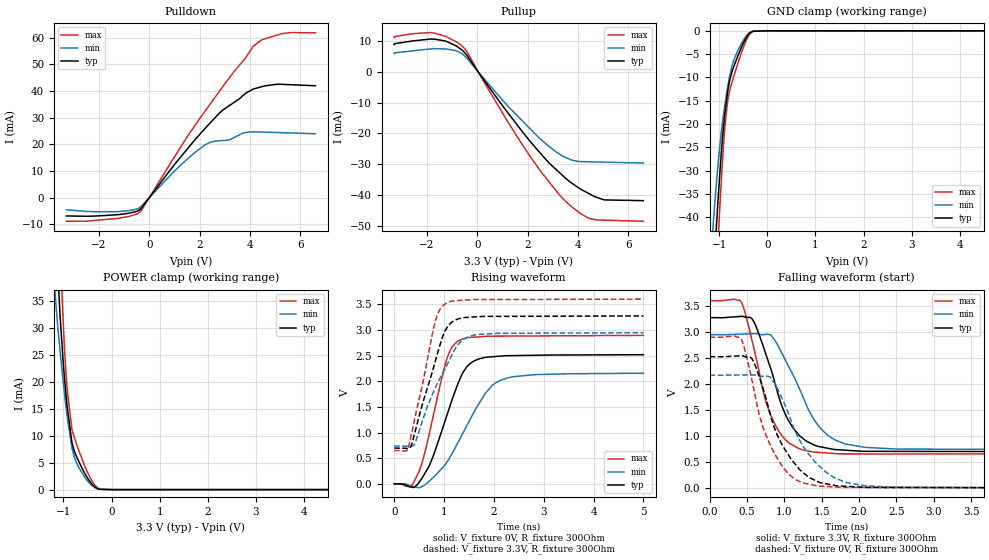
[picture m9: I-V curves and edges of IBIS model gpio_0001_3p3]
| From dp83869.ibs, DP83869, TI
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|   gpio_0001_3p3 Model
[Model]   gpio_0001_3p3
Model_type   I/O
Polarity   Non-Inverting
Enable   Active-Low
Vinl = 0.7
Vinh = 1.7
Vmeas = 1.65
Vref = 0
Cref = 2pF
Rref = 100000
|   typ   min   max
C_comp   1.10585pF   1.10585pF   1.45739pF
| Where Nom  PVT is Nominal Process, 3.3V,  27C
|   Fast PVT is Strong Process,  3.63V, -40C
|   Slow PVT is Weak Process,   2.97V, 125C
[Voltage Range]   3.3   2.97   3.63
|Junction Temperature
[Temperature Range]   27   125   -40
[Pullup Reference]   3.3   2.97   3.63
[Pulldown Reference]   -0   -0   -0
[Power Clamp Reference]   3.3   2.97   3.63
[GND Clamp Reference]   0   0   0
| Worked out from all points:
|   slope of the pulldown table from 0 to 0.495 V, typ, clamps not added: 79.9 ohm
|   slope of the pullup table from 0 to 0.495 V, typ, clamps not added: 87.3 ohm
|   GND clamp passes 1 mA (typ) near -0.41 V on its own axis
|   POWER clamp passes 1 mA (typ) near -0.41 V on its own axis
|   falling waveform, V_fixture 3.3V, R_fixture 300Ohm: 20-80 % time 382ps typ, 468ps min, 331ps max; typ from 3.27 V to 0.696 V
|   rising waveform, V_fixture 0V, R_fixture 300Ohm: 20-80 % time 538ps typ, 740ps min, 415ps max; typ from 0 V to 2.52 V
|   rising waveform, V_fixture 3.3V, R_fixture 300Ohm: 20-80 % time 464ps typ, 606ps min, 380ps max; typ from 0.696 V to 3.27 V
|   falling waveform, V_fixture 0V, R_fixture 300Ohm: 20-80 % time 426ps typ, 492ps min, 372ps max; typ from 2.52 V to 0 V
[Pulldown]
|   Voltage   I(typ)   I(min)   I(max)
-3.3V     -6.895mA   -4.586mA   -8.903mA
-1.256V   -6.433mA   -5.277mA   -7.816mA
-413.8mV  -4.752mA   -3.942mA   -5.716mA
1.117V    13.77mA    11.06mA    17.03mA
2.202V    25.82mA    19.71mA    32.27mA
2.893V    32.69mA    21.39mA    41.31mA
3.191V    34.6mA     21.69mA    45.1mA
3.723V    38.34mA    24.26mA    51.29mA
4.127V    40.73mA    24.68mA    56.79mA
4.47V     41.63mA    24.58mA    59.23mA
5.257V    42.5mA     24.35mA    61.51mA
6.6V      41.97mA    23.96mA    61.84mA
[GND Clamp]
|   Voltage   I(typ)   I(min)   I(max)
-3.3V     -489.2mA   -422.2mA   -556.8mA
-1.128V   -53.94mA   -41.75mA   -66.49mA
-1.053V   -40.94mA   -31.89mA   -50.85mA
-1.004V   -32.91mA   -26.23mA   -40.88mA
-914.8mV  -20.88mA   -18.15mA   -24.96mA
-886mV    -17.91mA   -16.01mA   -20.9mA
-824.7mV  -12.98mA   -11.96mA   -14.96mA
-737.5mV  -8.884mA   -7.637mA   -11.14mA
-632.6mV  -5.898mA   -4.664mA   -7.616mA
-450.4mV  -1.653mA   -1.242mA   -2.33mA
-360.4mV  -415.6uA   -340.7uA   -627.7uA
6.6V      0A         0A         0A
[Pullup]
|   Voltage   I(typ)   I(min)   I(max)
-3.3V     8.795mA    5.889mA    11.06mA
-1.778V   10.59mA    7.437mA    12.62mA
-1.241V   9.901mA    7.37mA     11.43mA
-595mV    6.955mA    5.791mA    8.28mA
-397mV    5.173mA    4.255mA    6.362mA
964.1mV   -10.58mA   -8.828mA   -12.86mA
1.883V    -20.4mA    -16.71mA   -24.79mA
2.688V    -28.11mA   -23.11mA   -34.04mA
3.438V    -34.02mA   -27.56mA   -41.45mA
4.426V    -39.49mA   -29.22mA   -47.53mA
5.047V    -41.59mA   -29.34mA   -48.14mA
6.6V      -41.83mA   -29.63mA   -48.52mA
[POWER Clamp]
|   Voltage   I(typ)   I(min)   I(max)
-3.3V     592.7mA    473.7mA    711.1mA
-1.183V   53.33mA    37.6mA     74.54mA
-1.164V   49.45mA    35.35mA    69.48mA
-1.121V   40.99mA    30.62mA    58.01mA
-1.071V   32.56mA    25.84mA    45.66mA
-1.013V   24.62mA    20.7mA     32.69mA
-952.4mV  18.17mA    15.83mA    22.43mA
-922.7mV  15.44mA    13.63mA    18.69mA
-824.7mV  8.834mA    7.855mA    11.3mA
-669.2mV  4.995mA    3.928mA    7.01mA
-332.6mV  387.6uA    312.9uA    668.4uA
6.6V      0A         0A         0A
[Ramp]
R_load = 300
|   typ   min   max
dV/dt_r   1.5107/5.36452e-10   1.29405/7.36382e-10   1.73698/4.12583e-10
dV/dt_f   1.5476/3.79865e-10   1.32601/4.6695e-10   1.77273/3.29959e-10
[Falling Waveform]
V_fixture = 3.3V
V_fixture_min = 2.97V
V_fixture_max = 3.63V
R_fixture = 300Ohm
C_fixture = 0F
|   Time   V(typ)   V(min)   V(max)
0s        3.275V     2.948V     3.603V
402.1ps   3.297V     2.956V     3.607V
569.5ps   3.25V      2.966V     2.82V
727.1ps   2.679V     2.948V     1.793V
816.1ps   2.298V     2.939V     1.401V
982.7ps   1.514V     2.545V     978.3mV
1.179ns   1.044V     1.983V     765.1mV
1.501ns   784.1mV    1.116V     678.1mV
1.834ns   723.2mV    839mV      653.8mV
5ns       695.9mV    737.6mV    648mV
[Rising Waveform]
V_fixture = 0V
V_fixture_min = 0V
V_fixture_max = 0V
R_fixture = 300Ohm
C_fixture = 0F
|   Time   V(typ)   V(min)   V(max)
0s        378.7uV    558.2uV    401.1uV
319.4ps   -58.11mV   -34.15mV   -57.08mV
486ps     13.86mV    -75.76mV   211mV
721.4ps   392.2mV    68.12mV    1.052V
1.045ns   1.299V     406.5mV    2.401V
1.291ns   1.977V     825.2mV    2.79V
1.608ns   2.4V       1.41V      2.861V
1.834ns   2.467V     1.769V     2.876V
2.146ns   2.492V     2.024V     2.881V
5ns       2.518V     2.157V     2.895V
[Rising Waveform]
V_fixture = 3.3V
V_fixture_min = 2.97V
V_fixture_max = 3.63V
R_fixture = 300Ohm
C_fixture = 0F
|   Time   V(typ)   V(min)   V(max)
0s        696mV      737.6mV    648mV
279.8ps   684.7mV    739.6mV    688.7mV
338.2ps   734.4mV    732mV      933.9mV
409.8ps   983.4mV    775.8mV    1.259V
816.1ps   2.361V     1.851V     3.139V
909.9ps   2.68V      2.041V     3.387V
1.033ns   3.002V     2.268V     3.517V
1.343ns   3.231V     2.781V     3.58V
1.682ns   3.259V     2.913V     3.594V
5ns       3.275V     2.947V     3.602V
[Falling Waveform]
|Gnd
V_fixture = 0V
V_fixture_min = 0V
V_fixture_max = 0V
R_fixture = 300Ohm
C_fixture = 0F
|   Time   V(typ)   V(min)   V(max)
0s        2.524V     2.166V     2.899V
419.1ps   2.541V     2.172V     2.871V
561.1ps   2.494V     2.174V     2.105V
667.3ps   2.121V     2.157V     1.387V
827.3ps   1.332V     2.105V     776.5mV
982.7ps   795.3mV    1.678V     395.9mV
1.229ns   319.6mV    852.6mV    104.8mV
1.551ns   80.57mV    307.3mV    27.51mV
2.086ns   10.73mV    40.29mV    7.631mV
5ns       370.8uV    533.6uV    395.3uV
